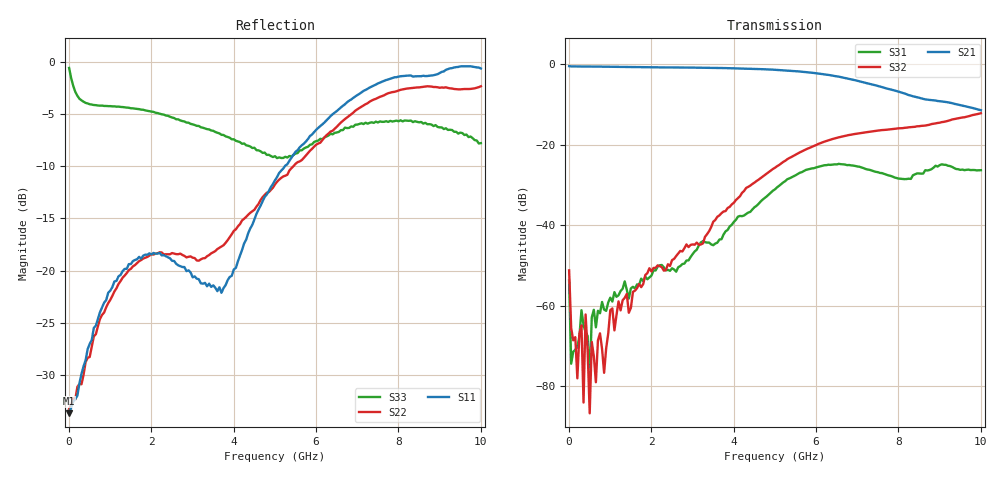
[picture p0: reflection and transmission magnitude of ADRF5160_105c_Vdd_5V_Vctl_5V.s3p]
!! Device:  ADRF5160
! Description: Silicon SPDT Switch
! Frequency:  0.7 -  4 GHz
! Ports:
!	RFc	= Port 1
!	RF1	= Port 2
!  RF2  = Port 3
! Vdd:  5 Volt
! Control:  5 Volt
! Data:  Data was collected using a calibrated 4 port network analyzer and de-embedded using Agilent's AFR De-Embedding.
! Note:  Analog Devices supplies this data as a sample of measured data
!  for this product.  Your particular data for this product may vary.
!  Data was taken at 105 degrees C.
!S3P File: Measurements: <S11,S12,S13>,
!<S21,S22,S23>,
!<S31,S32,S33>:
# Hz S  dB  R 50
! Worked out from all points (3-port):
!   201 points, 10 MHz to 10 GHz, reference 50 ohm
!   strongest paths, dB at 10 MHz, 2.507 GHz, 5.005 GHz, 7.503 GHz, 10 GHz:
!     S21: -0.5, -0.8, -1.4, -5.4, -11.4
!     S32: -51.3, -48.7, -25.8, -16.5, -12.2
!     S31: -53.8, -50.7, -31.1, -26.9, -26.4
!   lowest |S11| = -33.6 dB at 10 MHz (marker M1), VSWR 1.04, Z = 52.1 - j0.169 ohm
!   |S11| at or under -10 dB: start of sweep to 5.246 GHz
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1e7  -33.63 -4.5  -0.50 -0.1  -58.99 11.4
     -0.50 -0.5  -33.20 -15.1  -61.06 -16.9
     -53.77 34.0  -51.26 83.3  -0.61 -8.5
5.995e7  -33.08 -20.7  -0.59 -1.8  -65.90 -12.5
         -0.55 -1.6  -32.84 -13.6  -61.74 -4.2
         -74.48 122.4  -65.61 -65.4  -1.59 -45.3
2.098e8  -31.95 -43.9  -0.57 -5.5  -70.33 -6.5
         -0.57 -5.6  -31.10 -38.6  -74.89 -90.3
         -70.29 91.1  -78.10 57.6  -3.27 -110.2
3.097e8  -29.86 -54.3  -0.59 -8.1  -66.21 112.3
         -0.58 -8.1  -30.85 -55.9  -64.24 -126.3
         -61.17 78.2  -64.93 -123.1  -3.71 -131.7
3.5965e8  -29.13 -59.0  -0.58 -9.4  -70.48 66.1
          -0.58 -9.3  -29.95 -58.4  -71.32 15.1
          -64.85 83.4  -84.13 -44.2  -3.84 -138.8
4.096e8  -28.57 -66.0  -0.58 -10.7  -67.22 74.1
         -0.58 -10.6  -28.74 -65.4  -65.52 -117.5
         -66.64 60.3  -62.23 -135.4  -3.95 -145.3
5.095e8  -26.98 -70.5  -0.59 -13.3  -68.16 76.2
         -0.60 -13.2  -28.24 -75.4  -69.51 -108.5
         -78.44 157.2  -86.80 18.1  -4.09 -154.7
6.094e8  -25.46 -80.0  -0.60 -15.7  -61.83 76.8
         -0.60 -15.7  -26.27 -82.8  -70.22 -162.0
         -61.06 82.6  -72.57 158.9  -4.16 -161.9
5.005e9  -11.35 22.4  -1.41 -133.6  -30.97 94.8
         -1.41 -133.6  -11.74 -119.8  -25.74 118.9
         -31.12 95.0  -25.75 119.3  -9.05 104.6
1e10  -0.66 -65.9  -11.45 98.3  -26.29 -75.7
      -11.44 97.8  -2.36 84.1  -12.20 -72.3
      -26.35 -75.4  -12.20 -72.2  -7.80 10.8
